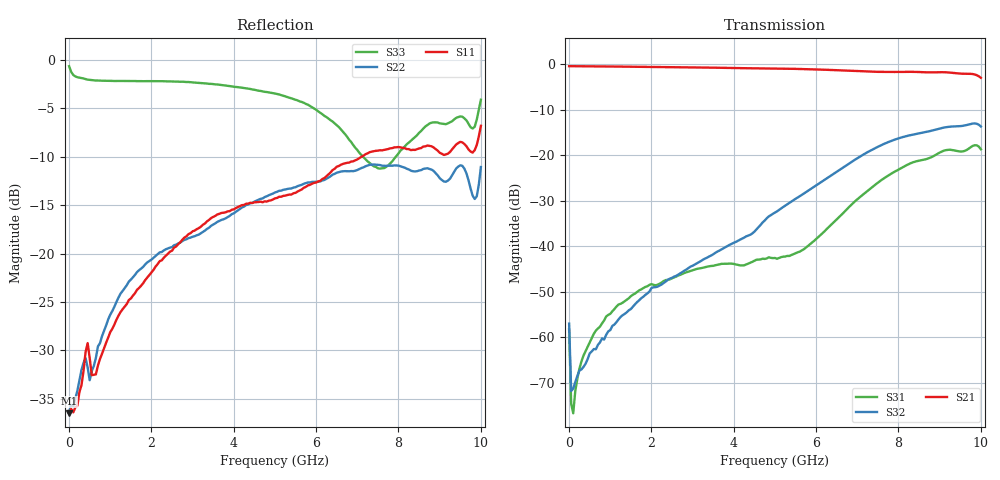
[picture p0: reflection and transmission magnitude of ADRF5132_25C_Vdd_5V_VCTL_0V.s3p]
! Device:  ADRF5132
! Description: Silicon SPDT Switch
! Frequency:  0.7 -  5 GHz
! Ports:
!	RFc	= Port 1
!	RF1	= Port 2
!  RF2  = Port 3
! Vdd:  5 Volt
! Control:  0/0 Volt
! Data:  Data was collected using a calibrated 4 port network analyzer and de-embedded using AtaiTec's In Situ De-Embedding.
! Note:  Analog Devices supplies this data as a sample of measured data
!  for this product.  Your particular data for this product may vary.
!  Data was taken at 25 degrees C.
!  Analog Devices reserves the right to change this data at anytime.
# GHZ S DB R 50.0
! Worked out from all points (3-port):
!   201 points, 10 MHz to 10 GHz, reference 50 ohm
!   strongest paths, dB at 10 MHz, 2.507 GHz, 5.005 GHz, 7.503 GHz, 10 GHz:
!     S21: -0.4, -0.6, -0.9, -1.6, -3.0
!     S32: -57.0, -47.0, -32.6, -18.1, -13.7
!     S31: -58.3, -47.1, -42.6, -26.0, -18.7
!   lowest |S11| = -36.5 dB at 10 MHz (marker M1), VSWR 1.03, Z = 51.4 + j0.512 ohm
!   |S11| at or under -10 dB: start of sweep to 7.101 GHz
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0.01  -36.49 19.4  -0.40 -0.2  -56.83 -62.6
      -0.40 -0.2  -36.28 22.7  -57.38 -55.5
      -58.30 -57.3  -57.04 -56.8  -0.64 -8.3
0.05995  -36.03 -12.3  -0.40 -1.0  -74.72 -48.3
         -0.40 -1.0  -35.63 -8.9  -72.25 -40.1
         -74.69 -44.2  -71.86 -37.3  -1.23 -42.3
0.1099  -36.39 -22.9  -0.40 -1.8  -75.48 26.8
        -0.41 -1.8  -35.78 -19.3  -71.42 -23.4
        -76.76 32.9  -71.33 -19.3  -1.55 -68.9
0.3097  -33.58 -43.1  -0.40 -5.0  -65.26 70.6
        -0.40 -5.0  -32.01 -41.0  -67.07 -44.5
        -65.33 73.3  -67.10 -42.7  -1.87 -127.5
0.65935  -32.47 -87.3  -0.45 -10.4  -58.45 79.4
         -0.45 -10.4  -30.77 -67.6  -62.60 -82.3
         -58.56 79.2  -62.67 -83.3  -2.12 -160.2
1.95805  -22.19 -127.3  -0.55 -30.4  -48.52 72.5
         -0.56 -30.4  -20.75 -104.0  -49.94 -139.1
         -48.52 72.5  -49.98 -139.4  -2.18 165.3
5.005  -14.29 156.8  -0.92 -77.0  -42.60 -3.1
       -0.93 -76.9  -13.68 -137.6  -32.59 -177.5
       -42.60 -3.0  -32.61 -177.4  -3.46 116.7
7.55245  -9.32 113.9  -1.65 -116.7  -25.67 179.1
         -1.65 -116.5  -10.85 -170.8  -17.89 114.8
         -25.69 179.4  -17.91 114.8  -11.22 111.1
9.6004  -8.68 71.4  -2.06 -151.6  -19.04 80.2
        -2.07 -151.2  -11.23 162.6  -13.45 41.2
        -19.05 80.5  -13.45 41.1  -6.03 100.6
10  -6.80 32.4  -2.95 -172.9  -18.66 29.3
    -2.96 -172.4  -11.05 116.7  -13.66 13.8
    -18.69 29.7  -13.67 13.7  -4.10 29.2
